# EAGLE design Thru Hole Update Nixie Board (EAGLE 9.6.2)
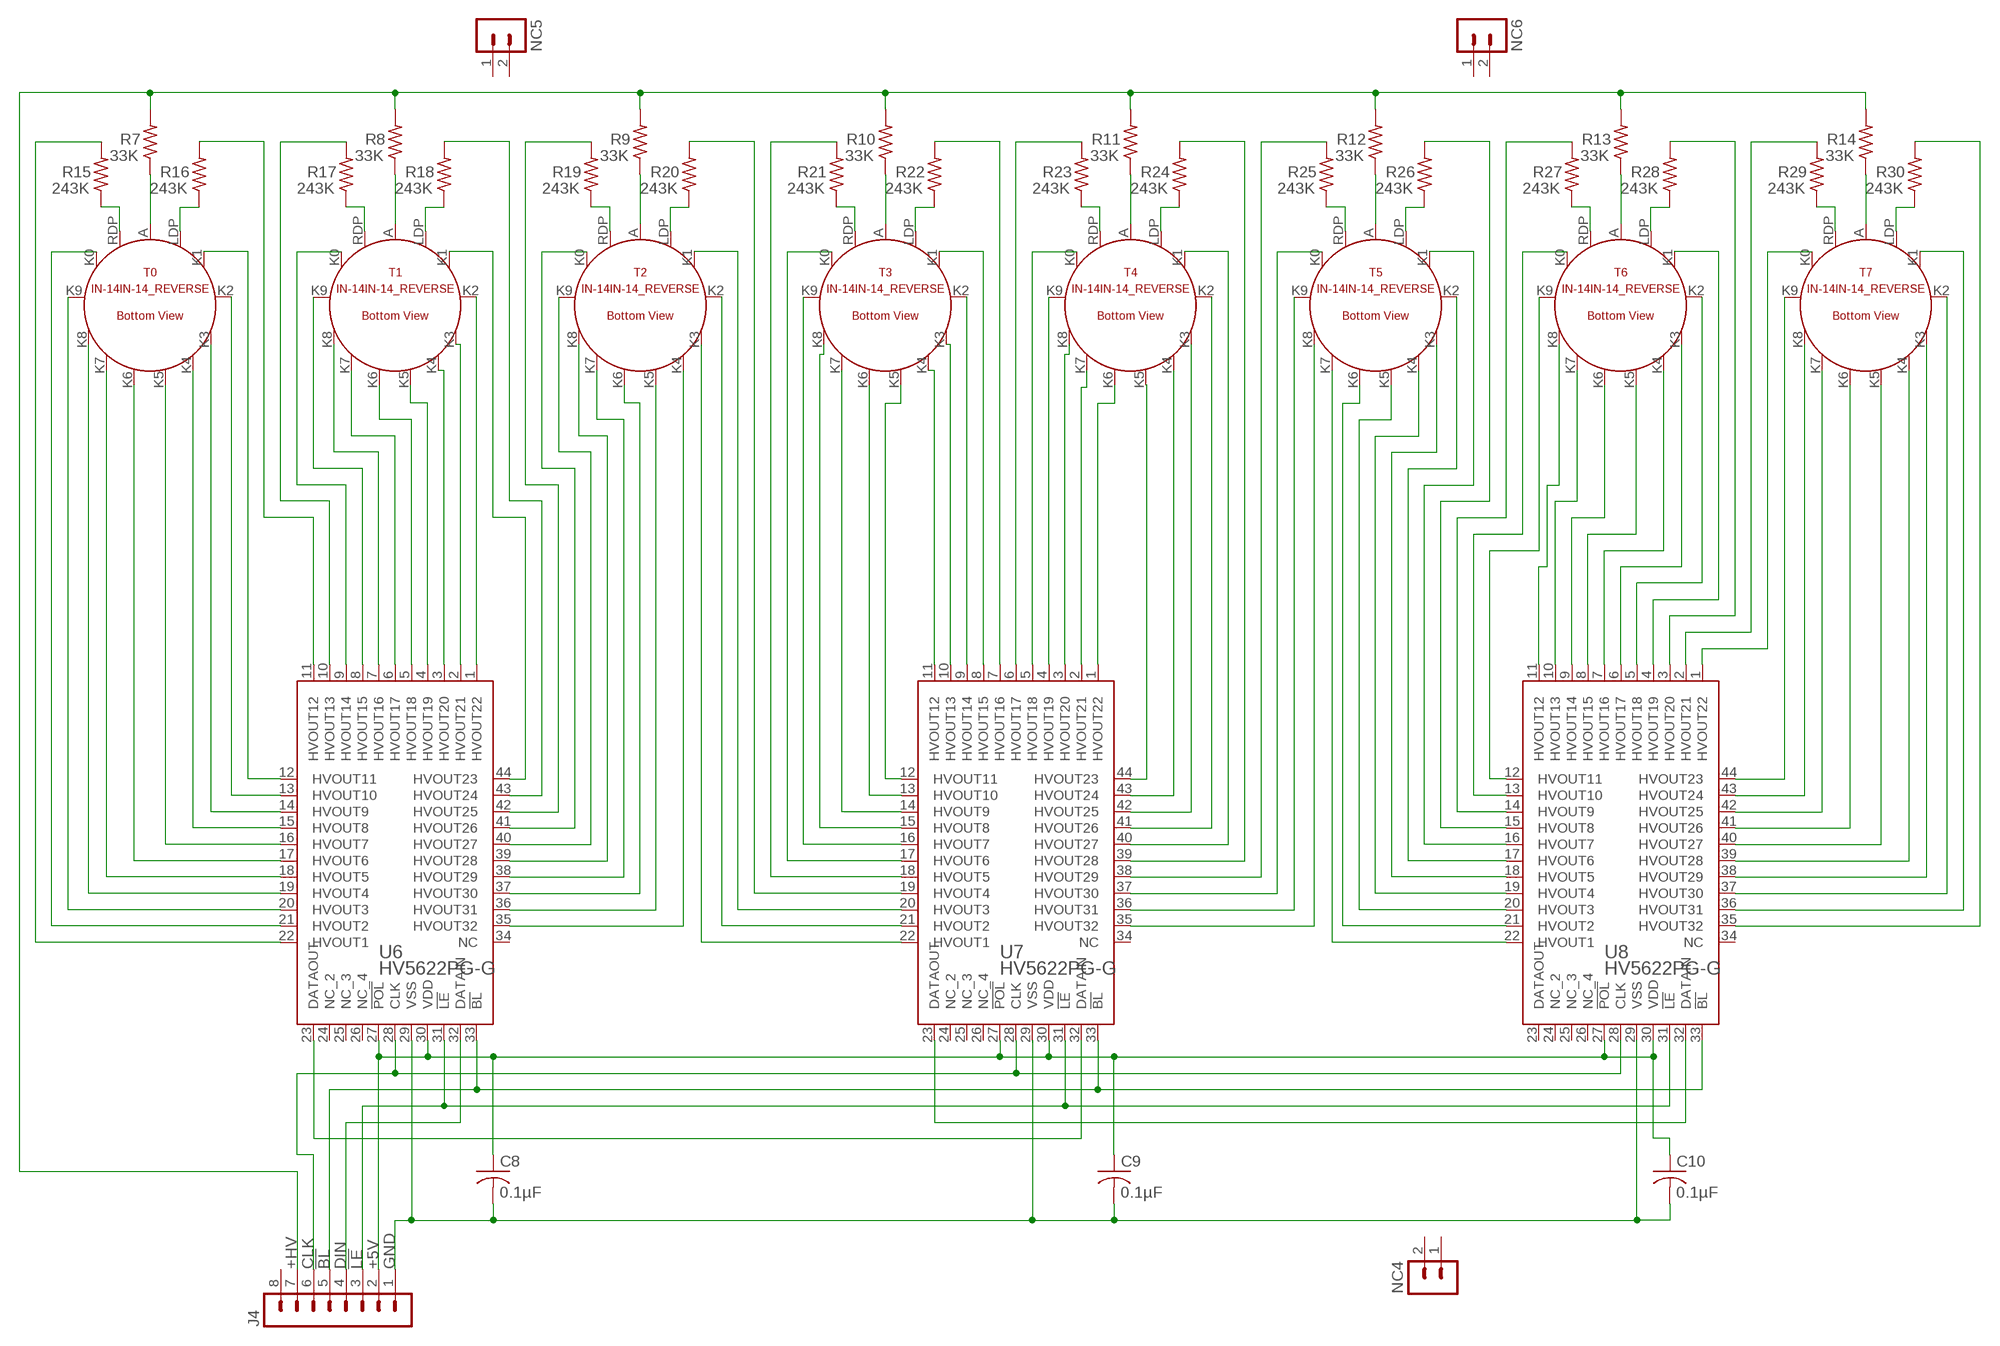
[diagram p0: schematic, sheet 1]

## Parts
C8  0.1µF  C-US  [C025-040X050]
C9  0.1µF  C-US  [C025-040X050]
C10  0.1µF  C-US  [C025-040X050]
J4  1  MA08  [MA08]
NC4  MA02  [MA02]
NC5  MA02  [MA02]
NC6  MA02  [MA02]
R7  33K  R-US0207/10  [0207/10]
R8  33K  R-US0207/10  [0207/10]
R9  33K  R-US0207/10  [0207/10]
R10  33K  R-US0207/10  [0207/10]
R11  33K  R-US0207/10  [0207/10]
R12  33K  R-US0207/10  [0207/10]
R13  33K  R-US0207/10  [0207/10]
R14  33K  R-US0207/10  [0207/10]
R15  243K  R-US0207/10  [0207/10]
R16  243K  R-US0207/10  [0207/10]
R17  243K  R-US0207/10  [0207/10]
R18  243K  R-US0207/10  [0207/10]
R19  243K  R-US0207/10  [0207/10]
R20  243K  R-US0207/10  [0207/10]
R21  243K  R-US0207/10  [0207/10]
R22  243K  R-US0207/10  [0207/10]
R23  243K  R-US0207/10  [0207/10]
R24  243K  R-US0207/10  [0207/10]
R25  243K  R-US0207/10  [0207/10]
R26  243K  R-US0207/10  [0207/10]
R27  243K  R-US0207/10  [0207/10]
R28  243K  R-US0207/10  [0207/10]
R29  243K  R-US0207/10  [0207/10]
R30  243K  R-US0207/10  [0207/10]
T0  IN-14IN-14_REVERSE  [IN-14_REVERSE]
T1  IN-14IN-14_REVERSE  [IN-14_REVERSE]
T2  IN-14IN-14_REVERSE  [IN-14_REVERSE]
T3  IN-14IN-14_REVERSE  [IN-14_REVERSE]
T4  IN-14IN-14_REVERSE  [IN-14_REVERSE]
T5  IN-14IN-14_REVERSE  [IN-14_REVERSE]
T6  IN-14IN-14_REVERSE  [IN-14_REVERSE]
T7  IN-14IN-14_REVERSE  [IN-14_REVERSE]
U6  HV5622PG-G  [QFP-44]
U7  HV5622PG-G  [QFP-44]
U8  HV5622PG-G  [QFP-44]

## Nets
!BL!: J4.5 U6.33(!BL) U7.33(!BL) U8.33(!BL)
!LE!: J4.3 U6.31(!LE) U7.31(!LE) U8.31(!LE)
+5V: C8.1 C9.1 C10.1 J4.2 U6.27(!POL) U6.30(VDD) U7.27(!POL) U7.30(VDD) U8.27(!POL) U8.30(VDD)
+HV: J4.7 R7.2 R8.2 R9.2 R10.2 R11.2 R12.2 R13.2 R14.2
CLK: J4.6 U6.28(CLK) U7.28(CLK) U8.28(CLK)
DIN: J4.4 U6.32(DATAIN)
GND: C8.2 C9.2 C10.2 J4.1 U6.29(VSS) U7.29(VSS) U8.29(VSS)
T0A: R7.1 T0.A
T1A: R8.1 T1.A
T2A: R9.1 T2.A
T3A: R10.1 T3.A
T4A: R11.1 T4.A
T5A: R12.1 T5.A
T6A: R13.1 T6.A
T7A: R14.1 T7.A
U5-T0K0: T0.K0 U6.21(HVOUT2)
U5-T0K1: T0.K1 U6.12(HVOUT11)
U5-T0K2: T0.K2 U6.13(HVOUT10)
U5-T0K3: T0.K3 U6.14(HVOUT9)
U5-T0K4: T0.K4 U6.15(HVOUT8)
U5-T0K5: T0.K5 U6.16(HVOUT7)
U5-T0K6: T0.K6 U6.17(HVOUT6)
U5-T0K7: T0.K7 U6.18(HVOUT5)
U5-T0K8: T0.K8 U6.19(HVOUT4)
U5-T0K9: T0.K9 U6.20(HVOUT3)
U5-T0LDP: R16.2 U6.11(HVOUT12)
U5-T0LDP1: R16.1 T0.LDP
U5-T0RDP: R15.2 U6.22(HVOUT1)
U5-T0RDP1: R15.1 T0.RDP
U5-T1K0: T1.K0 U6.9(HVOUT14)
U5-T1K1: T1.K1 U6.44(HVOUT23)
U5-T1K2: T1.K2 U6.1(HVOUT22)
U5-T1K3: T1.K3 U6.2(HVOUT21)
U5-T1K4: T1.K4 U6.3(HVOUT20)
U5-T1K5: T1.K5 U6.4(HVOUT19)
U5-T1K6: T1.K6 U6.5(HVOUT18)
U5-T1K7: T1.K7 U6.6(HVOUT17)
U5-T1K8: T1.K8 U6.7(HVOUT16)
U5-T1K9: T1.K9 U6.8(HVOUT15)
U5-T1LDP: R18.2 U6.43(HVOUT24)
U5-T1LDP1: R18.1 T1.LDP
U5-T1RDP: R17.2 U6.10(HVOUT13)
U5-T1RDP1: R17.1 T1.RDP
U5-T2K0: T2.K0 U6.41(HVOUT26)
U5-T2K4: T2.K4 U6.35(HVOUT32)
U5-T2K5: T2.K5 U6.36(HVOUT31)
U5-T2K6: T2.K6 U6.37(HVOUT30)
U5-T2K7: T2.K7 U6.38(HVOUT29)
U5-T2K8: T2.K8 U6.39(HVOUT28)
U5-T2K9: T2.K9 U6.40(HVOUT27)
U5-T2RDP: R19.2 U6.42(HVOUT25)
U5-T2RDP1: R19.1 T2.RDP
U5-U6: U6.23(DATAOUT) U7.32(DATAIN)
U6-T2K1: T2.K1 U7.20(HVOUT3)
U6-T2K2: T2.K2 U7.21(HVOUT2)
U6-T2K3: T2.K3 U7.22(HVOUT1)
U6-T2LDP: R20.2 U7.19(HVOUT4)
U6-T2LDP1: R20.1 T2.LDP
U6-T3K0: T3.K0 U7.17(HVOUT6)
U6-T3K1: T3.K1 U7.8(HVOUT15)
U6-T3K2: T3.K2 U7.9(HVOUT14)
U6-T3K3: T3.K3 U7.10(HVOUT13)
U6-T3K4: T3.K4 U7.11(HVOUT12)
U6-T3K5: T3.K5 U7.12(HVOUT11)
U6-T3K6: T3.K6 U7.13(HVOUT10)
U6-T3K7: T3.K7 U7.14(HVOUT9)
U6-T3K8: T3.K8 U7.15(HVOUT8)
U6-T3K9: T3.K9 U7.16(HVOUT7)
U6-T3LDP: R22.2 U7.7(HVOUT16)
U6-T3LDP1: R22.1 T3.LDP
U6-T3RDP: R21.2 U7.18(HVOUT5)
U6-T3RDP1: R21.1 T3.RDP
U6-T4K0: T4.K0 U7.5(HVOUT18)
U6-T4K1: T4.K1 U7.40(HVOUT27)
U6-T4K2: T4.K2 U7.41(HVOUT26)
U6-T4K3: T4.K3 U7.42(HVOUT25)
U6-T4K4: T4.K4 U7.43(HVOUT24)
U6-T4K5: T4.K5 U7.44(HVOUT23)
U6-T4K6: T4.K6 U7.1(HVOUT22)
U6-T4K7: T4.K7 U7.2(HVOUT21)
U6-T4K8: T4.K8 U7.3(HVOUT20)
U6-T4K9: T4.K9 U7.4(HVOUT19)
U6-T4LDP: R24.2 U7.39(HVOUT28)
U6-T4LDP1: R24.1 T4.LDP
U6-T4RDP: R23.2 U7.6(HVOUT17)
U6-T4RDP1: R23.1 T4.RDP
U6-T5K0: T5.K0 U7.37(HVOUT30)
U6-T5K8: T5.K8 U7.35(HVOUT32)
U6-T5K9: T5.K9 U7.36(HVOUT31)
U6-T5RDP: R25.2 U7.38(HVOUT29)
U6-T5RDP1: R25.1 T5.RDP
U6-U7: U7.23(DATAOUT) U8.32(DATAIN)
U7-T5K1: T5.K1 U8.16(HVOUT7)
U7-T5K2: T5.K2 U8.17(HVOUT6)
U7-T5K3: T5.K3 U8.18(HVOUT5)
U7-T5K4: T5.K4 U8.19(HVOUT4)
U7-T5K5: T5.K5 U8.20(HVOUT3)
U7-T5K6: T5.K6 U8.21(HVOUT2)
U7-T5K7: T5.K7 U8.22(HVOUT1)
U7-T5LDP: R26.2 U8.15(HVOUT8)
U7-T5LDP1: R26.1 T5.LDP
U7-T6K0: T6.K0 U8.13(HVOUT10)
U7-T6K1: T6.K1 U8.4(HVOUT19)
U7-T6K2: T6.K2 U8.5(HVOUT18)
U7-T6K3: T6.K3 U8.6(HVOUT17)
U7-T6K4: T6.K4 U8.7(HVOUT16)
U7-T6K5: T6.K5 U8.8(HVOUT15)
U7-T6K6: T6.K6 U8.9(HVOUT14)
U7-T6K7: T6.K7 U8.10(HVOUT13)
U7-T6K8: T6.K8 U8.11(HVOUT12)
U7-T6K9: T6.K9 U8.12(HVOUT11)
U7-T6LDP: R28.2 U8.3(HVOUT20)
U7-T6LDP1: R28.1 T6.LDP
U7-T6RDP: R27.2 U8.14(HVOUT9)
U7-T6RDP1: R27.1 T6.RDP
U7-T7K0: T7.K0 U8.1(HVOUT22)
U7-T7K1: T7.K1 U8.36(HVOUT31)
U7-T7K2: T7.K2 U8.37(HVOUT30)
U7-T7K3: T7.K3 U8.38(HVOUT29)
U7-T7K4: T7.K4 U8.39(HVOUT28)
U7-T7K5: T7.K5 U8.40(HVOUT27)
U7-T7K6: T7.K6 U8.41(HVOUT26)
U7-T7K7: T7.K7 U8.42(HVOUT25)
U7-T7K8: T7.K8 U8.43(HVOUT24)
U7-T7K9: T7.K9 U8.44(HVOUT23)
U7-T7LDP: R30.2 U8.35(HVOUT32)
U7-T7LDP1: R30.1 T7.LDP
U7-T7RDP: R29.2 U8.2(HVOUT21)
U7-T7RDP1: R29.1 T7.RDP
Unconnected: J4.8 NC4.1 NC4.2 NC5.1 NC5.2 NC6.1 NC6.2 U6.24(NC_2) U6.25(NC_3) U6.26(NC_4) U6.34(NC) U7.24(NC_2) U7.25(NC_3) U7.26(NC_4) U7.34(NC) U8.23(DATAOUT) U8.24(NC_2) U8.25(NC_3) U8.26(NC_4) U8.34(NC)

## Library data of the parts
C8-C10 = My Imported Components:C-US
J4 = My Imported Components:MA08: PIN HEADER; OC_FARNELL: unknown; OC_NEWARK: unknown
NC4-NC6 = My Imported Components:MA02: PIN HEADER
R7-R30 = My Imported Components:R-US: RESISTOR, American symbol; SPICEPREFIX: R
T0 T1-T7 = My Imported Components:IN-14
U6-U8 = My Imported Components:HV5622PG-G; BUILT_BY: EMA_Jessica; COPYRIGHT: Copyright (C) 2018 Accelerated Designs. All rights reserved; MANUFACTURER_PART_NUMBER: HV5622PG-G; SOURCELIBRARY: Microchip_2019-08-23_19; VENDOR: Microchip

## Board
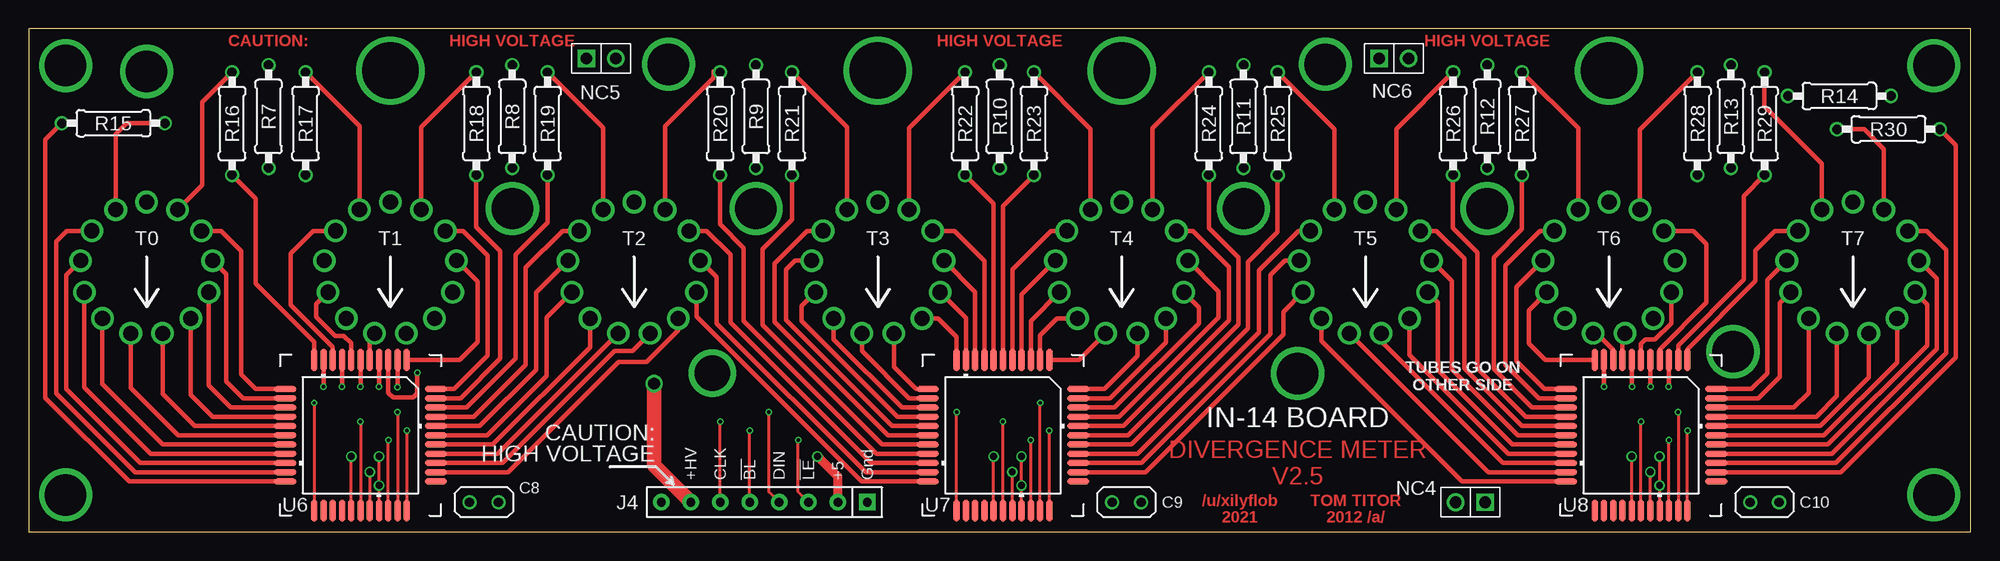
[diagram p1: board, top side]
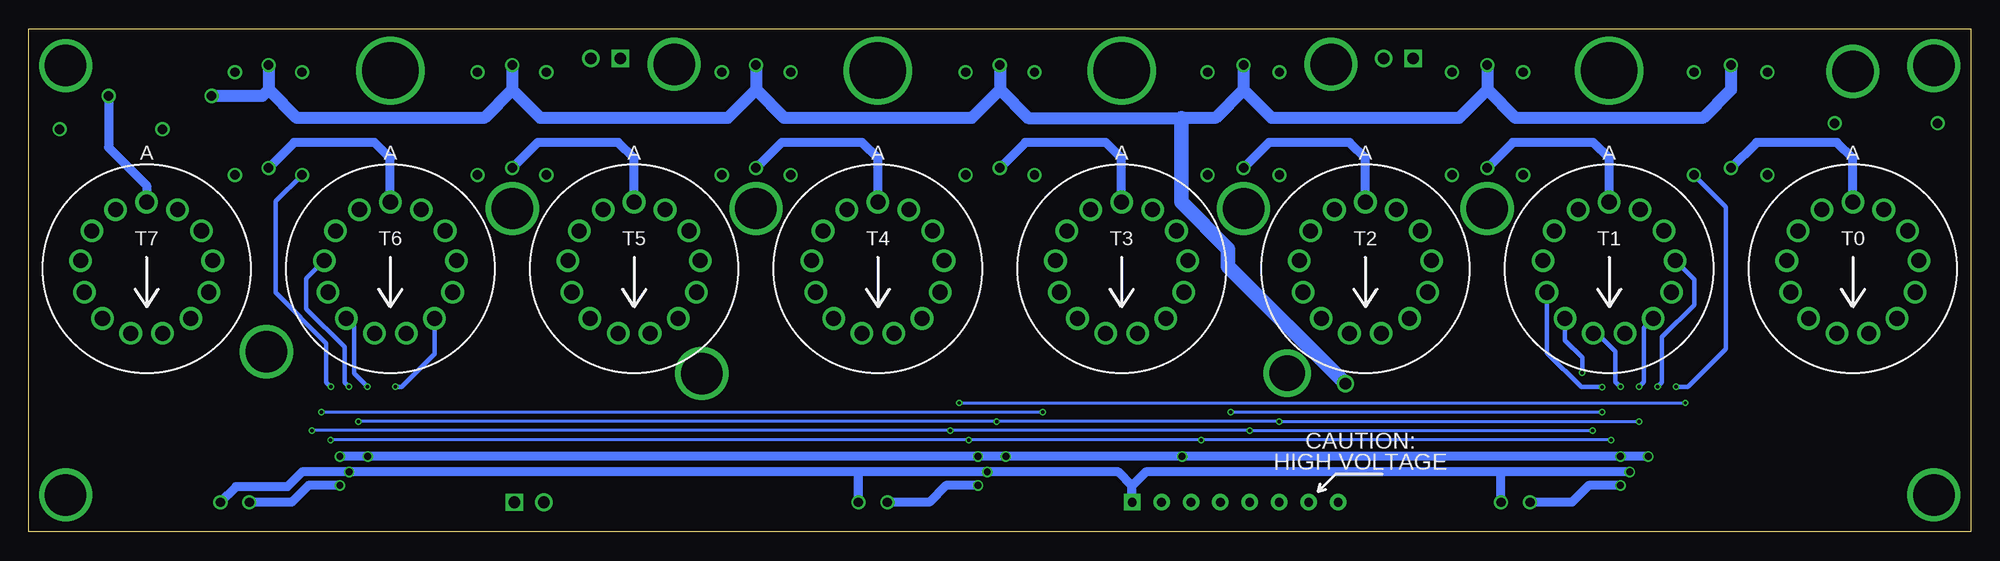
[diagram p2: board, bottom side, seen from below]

Size 167.64 x 43.43 mm. Coordinates in mm from the lower left corner, seen from the top.
Outline: 0,0 167.64,0 167.64,43.43 0,43.43 0,0
Copper layers (1*16): Top 0.035559375mm / dielectric 1.6mm / Bottom 0.035559375mm
Design rules "oshpark-2layer": minimum track width 6mil, minimum drill 10mil, track to track 6mil, track to pad 6mil, pad to pad 6mil, via to via 6mil, smd to smd 6mil, copper to edge 15mil, drill to drill 6mil, minimum pad ring 5mil, minimum via ring 5mil, stop-mask expansion 2.5mil, vias tented up to drill 0mil, thermal gap 10mil

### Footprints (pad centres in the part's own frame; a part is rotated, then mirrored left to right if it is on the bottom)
C025-040X050 = drill 0.813: 1 -1.25,0; 2 1.25,0
MA08 = drill 0.75 pad 1.422 square: 1 -8.89,0 | drill 0.75 pad 1.422: 2 -6.35,0; 3 -3.81,0; 4 -1.27,0; 5 1.27,0; 6 3.81,0; 7 6.35,0; 8 8.89,0
MA02 = drill 1 pad 1.422 square: 1 -1.27,0 | drill 1.016 pad 1.422: 2 1.27,0
0207/10 = drill 0.813: 1 -4.445,0; 2 4.445,0
IN-14_REVERSE = drill 1.3 pad 1.9: A 0,5.75; K0 4.732,3.266; K1 -4.732,3.266; K2 -5.708,0.693; K3 -5.376,-2.039; K4 -3.813,-4.304; K5 -1.376,-5.583; K6 1.376,-5.583; K7 3.813,-4.304; K8 5.376,-2.039; K9 5.708,0.693; LDP -2.672,5.091; RDP 2.672,5.091
QFP-44 = smd 1.9 x 0.55: 1 -6.5,4; 2 -6.5,3.2; 3 -6.5,2.4; 4 -6.5,1.6; 5 -6.5,0.8; 6 -6.5,0; 7 -6.5,-0.8; 8 -6.5,-1.6; 9 -6.5,-2.4; 10 -6.5,-3.2; 11 -6.5,-4; 23 6.5,-4; 24 6.5,-3.2; 25 6.5,-2.4; 26 6.5,-1.6; 27 6.5,-0.8; 28 6.5,0; 29 6.5,0.8; 30 6.5,1.6; 31 6.5,2.4; 32 6.5,3.2; 33 6.5,4 | smd 0.501 x 1.9: 12 -4,-6.5; 13 -3.2,-6.5; 14 -2.4,-6.5; 15 -1.6,-6.5; 16 -0.8,-6.5; 17 0,-6.5; 18 0.8,-6.5; 19 1.6,-6.5; 20 2.4,-6.5; 21 3.2,-6.5; 22 4,-6.5 | smd 0.55 x 1.9: 34 4,6.5; 35 3.2,6.5; 36 2.4,6.5; 37 1.6,6.5; 38 0.8,6.5; 39 0,6.5; 40 -0.8,6.5; 41 -1.6,6.5; 42 -2.4,6.5; 43 -3.2,6.5; 44 -4,6.5

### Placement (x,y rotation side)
C8  39.29,2.54 0 top
C9  94.77,2.54 0 top
C10  149.86,2.54 0 top
J4  63.5,2.54 180 top
NC4  124.46,2.54 180 top
NC5  49.4,40.89 0 top
NC6  117.86,40.89 0 top
R7  20.68,35.86 90 top
R8  41.73,35.86 90 top
R9  62.77,35.86 90 top
R10  83.82,35.86 90 top
R11  104.87,35.86 90 top
R12  125.91,35.86 90 top
R13  146.96,35.86 90 top
R14  156.31,37.64 180 top
R15  7.29,35.28 180 top
R16  17.53,35.26 270 top
R17  23.88,35.26 270 top
R18  38.63,35.26 270 top
R19  44.78,35.26 270 top
R20  59.68,35.26 270 top
R21  65.87,35.26 270 top
R22  80.82,35.26 270 top
R23  86.77,35.26 270 top
R24  101.87,35.26 270 top
R25  107.81,35.26 270 top
R26  122.97,35.26 270 top
R27  128.91,35.26 270 top
R28  144.06,35.26 270 top
R29  149.85,35.26 270 top
R30  160.55,34.77 0 top
T0  10.16,22.73 0 bottom
T1  31.21,22.73 0 bottom
T2  52.25,22.73 0 bottom
T3  73.3,22.73 0 bottom
T4  94.34,22.73 0 bottom
T5  115.39,22.73 0 bottom
T6  136.43,22.73 0 bottom
T7  157.48,22.73 0 bottom
U6  28.63,8.33 270 top
U7  84.1,8.33 270 top
U8  139.19,8.33 270 top

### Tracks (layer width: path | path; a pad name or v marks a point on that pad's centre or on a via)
!BL!  (via drill 0.3 pad 0.55)
  Top 0.254: v32.63,8.74 U6.33 | J4.5 v62.23,8.74 | U7.33 v88.1,8.74 | U8.33 v143.19,8.74
  Bottom 0.254: v32.63,8.74 v62.23,8.74 v88.1,8.74 v143.19,8.74
!LE!  (via drill 0.3 pad 0.55)
  Top 0.254: U6.31 v31.03,7.92 | U7.31 v86.5,7.92 | U8.31 v141.59,7.92 | J4.3 66.42,3.43 v66.42,7.92
  Bottom 0.254: v31.03,7.92 v66.42,7.92 v86.5,7.92 v141.59,7.92
+5V  (via drill 0.6 pad 0.8)
  Top 0.254: U6.27 v27.83,6.5 | U6.30 v30.23,3.99 v30.23,6.5 | U7.30 v85.7,3.99 v85.7,6.5 | U7.27 v83.3,6.5 | U8.30 v140.79,3.99 v140.79,6.5 | U8.27 v138.39,6.5
  Top 0.762: J4.2 69.85,4.72 v68.07,6.5
  Bottom 0.762: v27.83,6.5 v30.23,6.5 v68.07,6.5 v83.3,6.5 v85.7,6.5 v138.39,6.5 v140.79,6.5 | v140.79,3.99 143.51,3.99 144.96,2.54 C10.1 | C9.1 89.89,2.54 88.44,3.99 v85.7,3.99 | v30.23,3.99 32.97,3.99 34.42,2.54 C8.1
+HV  (via drill 1 pad 1.5)
  Top 1.27: v53.98,12.8 53.98,5.71 J4.7
  Bottom 1.016: R7.2 20.68,38.18 23.12,35.74 39.29,35.74 41.73,38.18 | R8.2 41.73,38.18 | 41.73,38.18 44.17,35.74 60.34,35.74 62.77,38.18 | R9.2 62.77,38.18 | R10.2 83.82,38.18 | R11.2 104.87,38.18 | R12.2 125.91,38.18 | R13.2 146.96,38.18 | 146.96,38.18 144.52,35.74 128.35,35.74 125.91,38.18 | 125.91,38.18 123.47,35.74 107.3,35.74 104.87,38.18 | 104.87,38.18 102.43,35.74 86.26,35.74 83.82,38.18 | 83.82,38.18 81.38,35.74 68.15,35.74 65.21,35.74 62.77,38.18 | 146.96,38.18 147.49,37.64 R14.2
  Bottom 1.27: v53.98,12.8 64.11,22.91 64.11,24.43 68.15,28.5 68.15,35.74
CLK  (via drill 0.3 pad 0.55)
  Top 0.254: v28.63,9.53 U6.28 | J4.6 v59.69,9.53 | U7.28 v84.1,9.53 | U8.28 v139.19,9.53
  Bottom 0.254: v28.63,9.53 v59.69,9.53 v84.1,9.53 v139.19,9.53
DIN  (via drill 0.3 pad 0.55)
  Top 0.254: v31.83,10.34 U6.32 | J4.4 63.88,3.43 v63.88,10.34
  Bottom 0.254: v63.88,10.34 v31.83,10.34
GND  (via drill 0.6 pad 0.8)
  Top 0.254: v29.43,5.16 U6.29 | U7.29 v84.9,5.16 | U8.29 v139.99,5.16
  Bottom 0.762: v29.43,5.16 40.54,5.16 | 40.54,5.16 71.2,5.16 72.39,3.96 | 96.01,5.16 v84.9,5.16 73.58,5.16 72.39,3.96 | 96.01,5.16 v139.99,5.16 144.07,5.16 145.34,3.89 149.76,3.89 C10.2 | C9.2 96.02,5.15 96.01,5.16 | C8.2 40.54,5.15 40.54,5.16 | J4.1 72.39,3.96
N$1  (via drill 3.05 pad 3.48)
  other vias: 59,13.69
N$2  (via drill 3.58 pad 4.01)
  other vias: 55.22,40.39
N$3  (via drill 3.58 pad 4.01)
  other vias: 104.87,27.91
N$4  (via drill 3.58 pad 4.01)
  other vias: 62.77,27.91
N$5  (via drill 3.58 pad 4.01)
  other vias: 10.16,39.75
N$6  (via drill 3.58 pad 4.01)
  other vias: 109.55,13.67
N$7  (via drill 3.58 pad 4.01)
  other vias: 111.94,40.39
N$8  (via drill 3.58 pad 4.01)
  other vias: 41.73,27.91
N$9  (via drill 3.58 pad 4.01)
  other vias: 147.14,15.54
N$10  (via drill 3.58 pad 4.27)
  other vias: 3.17,3.17
N$11  (via drill 3.58 pad 4.27)
  other vias: 164.47,3.17
N$12  (via drill 3.58 pad 4.27)
  other vias: 3.17,40.26
N$13  (via drill 3.58 pad 4.27)
  other vias: 164.47,40.26
N$14  (via drill 4.88 pad 5.59)
  other vias: 73.3,39.83
N$15  (via drill 4.88 pad 5.59)
  other vias: 94.34,39.83
N$16  (via drill 4.88 pad 5.59)
  other vias: 136.43,39.83
N$17  (via drill 4.88 pad 5.59)
  other vias: 31.21,39.83
N$18  (via drill 3.58 pad 4.01)
  other vias: 125.91,27.91
T0A
  Bottom 0.762: T0.A 10.16,32.26 11.53,33.63 18.47,33.63 R7.1
T1A
  Bottom 0.762: T1.A 31.21,32.26 32.58,33.63 39.52,33.63 R8.1
T2A
  Bottom 0.762: T2.A 52.25,32.26 53.62,33.63 60.56,33.63 R9.1
T3A
  Bottom 0.762: T3.A 73.3,32.26 74.67,33.63 81.61,33.63 R10.1
T4A
  Bottom 0.762: T4.A 94.34,32.26 95.71,33.63 102.66,33.63 R11.1
T5A
  Bottom 0.762: T5.A 115.39,32.26 116.76,33.63 123.7,33.63 R12.1
T6A
  Bottom 0.762: T6.A 136.43,32.26 137.81,33.63 144.75,33.63 R13.1
T7A
  Bottom 0.762: T7.A 157.48,29.92 160.76,33.2 R14.1
U5-T0K0
  Top 0.381: U6.21 9.17,5.13 2.34,11.96 2.34,25.08 3.25,25.99 T0.K0
U5-T0K1
  Top 0.381: U6.12 19.58,12.33 18.31,13.6 18.31,24.26 16.58,25.99 T0.K1
U5-T0K2
  Top 0.381: U6.13 18.48,11.53 17.04,12.97 17.04,22.24 T0.K2
U5-T0K3
  Top 0.381: U6.14 17.43,10.73 15.54,12.62 T0.K3
U5-T0K4
  Top 0.381: U6.15 15.88,9.93 13.97,11.84 T0.K4
U5-T0K5
  Top 0.381: U6.16 14.29,9.13 11.54,11.89 T0.K5
U5-T0K6
  Top 0.381: U6.17 12.87,8.33 8.78,12.42 T0.K6
U5-T0K7
  Top 0.381: U6.18 11.57,7.53 6.35,12.75 T0.K7
U5-T0K8
  Top 0.381: U6.19 10.5,6.73 4.78,12.45 T0.K8
U5-T0K9
  Top 0.381: U6.20 9.61,5.93 3.23,12.32 3.23,22.19 T0.K9
U5-T0LDP
  Top 0.381: U6.11 24.63,16.39 19.58,21.44 19.58,28.76 R16.2
U5-T0LDP1
  Top 0.381: T0.LDP 14.96,29.95 14.96,37.13 R16.1
U5-T0RDP
  Top 0.381: U6.22 8.65,4.33 1.42,11.56 1.42,33.86 R15.2
U5-T0RDP1
  Top 0.381: T0.RDP 7.49,34.34 8.43,35.28 R15.1
U5-T1K0
  Top 0.381: U6.9 26.23,15.95 22.59,19.58 22.59,24.03 24.56,25.99 T1.K0
U5-T1K1
  Top 0.381: U6.44 36.73,12.33 39.61,15.21 39.61,23.85 37.47,25.99 T1.K1
U5-T1K2
  Top 0.381: U6.1 37.17,14.83 38.72,16.38 38.72,21.61 T1.K2
U5-T1K3  (via drill 0.3 pad 0.55)
  Top 0.381: U6.2 v31.83,12.5
  Bottom 0.381: v31.83,12.5 33.62,12.5 36.58,15.46 T1.K3
U5-T1K4  (via drill 0.3 pad 0.55)
  Top 0.381: U6.3 31.03,12 31.45,11.58 33.17,11.58 33.53,11.94 v33.53,13.74
  Bottom 0.381: v33.53,13.74 33.53,15.04 35.02,16.53 T1.K4
U5-T1K5  (via drill 0.3 pad 0.55)
  Top 0.381: U6.4 v30.23,12.52
  Bottom 0.381: v30.23,12.52 30.65,12.94 30.65,15.56 32.23,17.14 T1.K5
U5-T1K6
  Top 0.381: U6.5 29.43,16.74 T1.K6
U5-T1K7  (via drill 0.3 pad 0.55)
  Top 0.381: U6.6 v28.63,12.52
  Bottom 0.381: v28.63,12.52 28.21,12.94 28.21,17.61 T1.K7
U5-T1K8
  Top 0.381: U6.7 27.83,16.28 27.19,16.92 26.43,16.92 24.8,18.54 24.8,19.66 T1.K8
U5-T1K9  (via drill 0.3 pad 0.55)
  Top 0.381: U6.8 v27.03,12.52
  Bottom 0.381: v27.03,12.52 26.63,12.91 26.63,16.82 23.86,19.58 23.86,21.79 T1.K9
U5-T1LDP
  Top 0.381: U6.43 37.26,11.53 40.69,14.96 40.69,24.25 38.63,26.31 R18.2
U5-T1LDP1
  Top 0.381: T1.LDP 33.88,34.95 R18.1
U5-T1RDP  (via drill 0.3 pad 0.55)
  Top 0.381: U6.10 v25.43,12.52
  Bottom 0.381: v25.43,12.52 24.41,12.52 21.13,15.8 21.13,28.06 R17.2
U5-T1RDP1
  Top 0.381: T1.RDP 28.53,35.05 R17.1
U5-T2K0
  Top 0.381: U6.41 38.38,9.93 42.88,14.43 42.88,22.81 46.06,25.99 T2.K0
U5-T2K4
  Top 0.381: U6.35 41.38,5.13 50.91,14.66 53.32,14.66 56.06,17.4 T2.K4
U5-T2K5
  Top 0.381: U6.36 40.88,5.93 50.58,15.62 52.11,15.62 T2.K5
U5-T2K6
  Top 0.381: U6.37 40.46,6.73 T2.K6
U5-T2K7
  Top 0.381: U6.38 40.05,7.53 48.44,15.92 T2.K7
U5-T2K8
  Top 0.381: U6.39 39.58,8.33 44.68,13.44 44.68,18.49 T2.K8
U5-T2K9
  Top 0.381: U6.40 38.93,9.13 43.77,13.97 43.77,20.64 T2.K9
U5-T2RDP
  Top 0.381: U6.42 37.78,10.73 42.04,14.99 42.04,23.96 44.78,26.7 R19.2
U5-T2RDP1
  Top 0.381: R19.1 49.58,34.9 T2.RDP
U5-U6  (via drill 0.3 pad 0.55)
  Top 0.254: v24.63,11.12 U6.23 | U7.32 v87.3,11.12
  Bottom 0.254: v87.3,11.12 v24.63,11.12
U6-T2K1
  Top 0.381: U7.20 72.71,5.93 60.58,18.06 60.58,23.93 58.52,25.99 T2.K1
U6-T2K2
  Top 0.381: U7.21 72.27,5.13 59.39,18.01 59.39,21.99 T2.K2
U6-T2K3
  Top 0.381: U7.22 71.87,4.33 57.63,18.58 T2.K3
U6-T2LDP
  Top 0.381: U7.19 73.2,6.73 61.72,18.21 61.72,24.51 59.67,26.56 R20.2
U6-T2LDP1
  Top 0.381: R20.1 59.13,39.79 59.13,39.23 54.92,35.02 T2.LDP
U6-T3K0
  Top 0.381: U7.17 74.16,8.33 64.36,18.14 64.36,23.16 67.18,25.99 T3.K0
U6-T3K1
  Top 0.381: U7.8 82.5,23.39 79.89,25.99 T3.K1
U6-T3K2
  Top 0.381: U7.9 81.7,20.72 T3.K2
U6-T3K3
  Top 0.381: U7.10 80.9,18.46 T3.K3
U6-T3K4
  Top 0.381: U7.11 80.1,16.82 78.5,18.42 T3.K4
U6-T3K5
  Top 0.381: U7.12 76.59,12.33 74.67,14.24 T3.K5
U6-T3K6
  Top 0.381: U7.13 75.99,11.53 71.92,15.6 T3.K6
U6-T3K7
  Top 0.381: U7.14 75.37,10.73 69.48,16.61 T3.K7
U6-T3K8
  Top 0.381: U7.15 75,9.93 66.72,18.21 66.72,19.48 T3.K8
U6-T3K9
  Top 0.381: U7.16 74.53,9.13 65.37,18.29 65.37,22.66 66.13,23.42 T3.K9
U6-T3LDP
  Top 0.381: R22.2 83.3,28.33 U7.7
U6-T3LDP1
  Top 0.381: R22.1 75.97,34.85 T3.LDP
U6-T3RDP
  Top 0.381: U7.18 73.65,7.53 63.32,17.86 63.32,24.42 65.87,26.98 R21.2
U6-T3RDP1
  Top 0.381: R21.1 70.62,34.95 T3.RDP
U6-T4K0
  Top 0.381: U7.5 84.9,22.66 88.23,25.99 T4.K0
U6-T4K1
  Top 0.381: U7.40 94.51,9.13 103.61,18.24 103.61,22.89 100.51,25.99 T4.K1
U6-T4K2
  Top 0.381: U7.41 94.11,9.93 102.7,18.52 102.7,20.77 T4.K2
U6-T4K3
  Top 0.381: U7.42 93.75,10.73 101.02,18.01 101.02,19.38 T4.K3
U6-T4K4
  Top 0.381: U7.43 93.35,11.53 98.16,16.34 T4.K4
U6-T4K5
  Top 0.381: U7.44 92.86,12.33 95.72,15.19 T4.K5
U6-T4K6
  Top 0.381: U7.1 90.66,14.83 T4.K6
U6-T4K7
  Top 0.381: U7.2 87.3,16.96 88.76,18.42 T4.K7
U6-T4K8
  Top 0.381: U7.3 86.5,18.22 T4.K8
U6-T4K9
  Top 0.381: U7.4 85.7,20.48 T4.K9
U6-T4LDP
  Top 0.381: U7.39 94.87,8.33 104.42,17.88 104.42,23.69 101.87,26.24 R24.2
U6-T4LDP1
  Top 0.381: R24.1 97.02,34.85 T4.LDP
U6-T4RDP
  Top 0.381: R23.2 84.1,28.14 U7.6
U6-T4RDP1
  Top 0.381: R23.1 91.67,34.8 T4.RDP
U6-T5K0
  Top 0.381: U7.37 95.7,6.73 106.19,17.22 106.19,22.58 109.61,25.99 T5.K0
U6-T5K8
  Top 0.381: U7.35 96.42,5.13 108.33,17.04 108.33,19 T5.K8
U6-T5K9
  Top 0.381: U7.36 96.07,5.93 107.21,17.07 107.21,22.17 108.45,23.42 T5.K9
U6-T5RDP
  Top 0.381: U7.38 95.21,7.53 105.26,17.58 105.26,23.32 107.81,25.87 R25.2
U6-T5RDP1
  Top 0.381: R25.1 112.72,34.8 T5.RDP
U6-U7  (via drill 0.3 pad 0.55)
  Top 0.254: U7.23 v80.1,10.34 | v142.39,10.34 U8.32
  Bottom 0.254: v142.39,10.34 v80.1,10.34
U7-T5K1
  Top 0.381: U8.16 128.91,9.13 123.92,14.12 123.92,23.6 121.53,25.99 T5.K1
U7-T5K2
  Top 0.381: U8.17 128.55,8.33 122.86,14.02 122.86,21.66 T5.K2
U7-T5K3
  Top 0.381: U8.18 128.1,7.53 121.64,13.99 121.64,19.82 T5.K3
U7-T5K4
  Top 0.381: U8.19 127.73,6.73 119.2,15.26 T5.K4
U7-T5K5
  Top 0.381: U8.20 127.26,5.93 116.77,16.43 T5.K5
U7-T5K6
  Top 0.381: U8.21 126.02,5.13 T5.K6
U7-T5K7
  Top 0.381: U8.22 123.71,4.33 111.58,16.46 T5.K7
U7-T5LDP
  Top 0.381: U8.15 129.26,9.93 125.07,14.12 125.07,24.11 122.97,26.21 R26.2
U7-T5LDP1
  Top 0.381: R26.1 118.06,34.8 T5.LDP
U7-T6K0
  Top 0.381: U8.13 130.36,11.53 127.47,14.43 127.47,22.99 130.47,25.99 T6.K0
U7-T6K1
  Top 0.381: U8.4 140.79,15.74 144.84,19.79 144.84,24.87 143.72,25.99 T6.K1
U7-T6K2  (via drill 0.3 pad 0.55)
  Top 0.381: U8.5 139.99,12.54 v140,12.52
  Bottom 0.381: v140,12.52 140.4,12.91 140.4,15.95 143.7,19.25 143.7,21.86 T6.K2
U7-T6K3
  Top 0.381: U8.6 139.19,16.23 139.55,16.59 140.39,16.59 141.81,18.01 T6.K3
U7-T6K4  (via drill 0.3 pad 0.55)
  Top 0.381: U8.7 138.39,12.54 v138.41,12.52
  Bottom 0.381: v138.41,12.52 139.56,13.68 139.56,17.73 T6.K4
U7-T6K5
  Top 0.381: U8.8 137.59,16.92 T6.K5
U7-T6K6
  Top 0.381: U8.9 136.79,15.72 135.37,17.14 T6.K6
U7-T6K7  (via drill 0.3 pad 0.55)
  Top 0.381: U8.10 v135.99,12.52
  Bottom 0.381: T6.K7 132.62,15.37 135.47,12.52 v135.99,12.52
U7-T6K8
  Top 0.381: U8.11 130.95,14.83 129.5,16.28 129.5,19.13 T6.K8
U7-T6K9
  Top 0.381: U8.12 130.86,12.33 128.43,14.76 128.43,21.12 T6.K9
U7-T6LDP  (via drill 0.3 pad 0.55)
  Top 0.381: U8.3 141.59,12.54 v141.58,12.52
  Bottom 0.381: v141.58,12.52 141.96,12.9 141.96,16.28 146.33,20.65 146.33,28.54 R28.2
U7-T6LDP1
  Top 0.381: R28.1 139.11,34.74 T6.LDP
U7-T6RDP
  Top 0.381: U8.14 129.78,10.73 126.47,14.05 126.47,23.7 128.91,26.14 R27.2
U7-T6RDP1
  Top 0.381: R27.1 133.76,34.85 T6.RDP
U7-T7K0
  Top 0.381: U8.1 143.19,15.76 149.07,21.64 149.07,24.31 150.76,25.99 T7.K0
U7-T7K1
  Top 0.381: U8.36 156.02,5.93 165.53,15.44 165.53,24.33 163.87,25.99 T7.K1
U7-T7K2
  Top 0.381: U8.37 155.68,6.73 164.72,15.77 164.72,21.89 T7.K2
U7-T7K3
  Top 0.381: U8.38 155.33,7.53 163.91,16.1 163.91,19.64 T7.K3
U7-T7K4
  Top 0.381: U8.39 154.99,8.33 161.29,14.63 T7.K4
U7-T7K5
  Top 0.381: T7.K5 158.86,13.34 154.65,9.13 U8.40
U7-T7K6
  Top 0.381: U8.41 154.31,9.93 156.1,11.73 T7.K6
U7-T7K7
  Top 0.381: U8.42 152.4,10.73 153.67,12 T7.K7
U7-T7K8
  Top 0.381: U8.43 149.3,11.53 151.16,13.39 151.16,19.74 T7.K8
U7-T7K9
  Top 0.381: U8.44 148.73,12.33 150.09,13.69 150.09,21.73 T7.K9
U7-T7LDP
  Top 0.381: U8.35 156.44,5.13 166.37,15.06 166.37,33.4 R30.2
U7-T7LDP1
  Top 0.381: T7.LDP 160.15,33.07 158.44,34.77 R30.1
U7-T7RDP
  Top 0.381: U8.2 142.39,16.1 148.06,21.77 148.06,29.01 R29.2
U7-T7RDP1
  Top 0.381: T7.RDP 154.81,31.8 149.85,36.75 R29.1

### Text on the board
Top: CAUTION: | HIGH VOLTAGE | HIGH VOLTAGE | HIGH VOLTAGE | DIVERGENCE METER / V2.5 | /u/xilyflob / 2021 | TOM TITOR / 2012 /a/
tPlace: T0 | T1 | T2 | T3 | T4 | T5 | T6 | T7 | TUBES GO ON / OTHER SIDE | IN-14 BOARD | CAUTION: / HIGH VOLTAGE | +HV | CLK | !BL! | DIN | !LE! | +5 | Gnd
bPlace: CAUTION: / HIGH VOLTAGE
tStop: CAUTION: | HIGH VOLTAGE | HIGH VOLTAGE | HIGH VOLTAGE | DIVERGENCE METER / V2.5 | /u/xilyflob / 2021 | TOM TITOR / 2012 /a/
